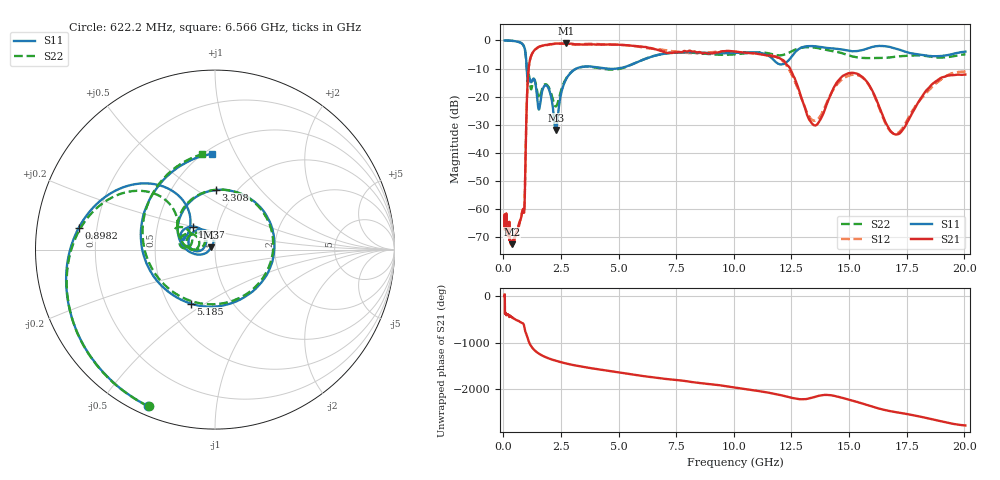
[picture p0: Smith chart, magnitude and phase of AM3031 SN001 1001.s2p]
# Hz S DB R 50
!freq MagS11 AngS11 MagS21 AngS21 MagS12 AngS12 MagS22 AngS22
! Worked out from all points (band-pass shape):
!   1601 points, 50 MHz to 20.05 GHz, reference 50 ohm
!   highest |S21| = -1.05 dB at 2.702 GHz (marker M1); lowest = -72.5 dB at 372.4 MHz (marker M2)
!   |S21| within 3 dB of the highest: 1.292 GHz to 6.925 GHz (5.633 GHz wide, 137 % of centre); 9.395 GHz to 10.15 GHz (758.8 MHz wide, 7.76 % of centre)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
!   lowest |S11| = -31.9 dB at 2.274 GHz (marker M3), VSWR 1.05, Z = 47.9 + j1.31 ohm
!   |S11| at or under -10 dB: 1.01 GHz to 3.165 GHz (2.155 GHz wide, 103 % of centre); 4.463 GHz to 4.928 GHz (464.8 MHz wide, 9.9 % of centre)
!   |S22| runs from -23.5 to 0.0 dB; largest |S21 - S12| = 0.067
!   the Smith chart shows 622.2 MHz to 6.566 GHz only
!   S11 on the Smith chart (normalised r, x): 622.2 MHz: 0.04, -0.66; 898.2 MHz: 0.13, +0.08; 1.377 GHz: 0.75, +0.20; 3.308 GHz: 0.81, +0.60; 5.185 GHz: 0.65, -0.44; 6.566 GHz: 0.54, +0.81
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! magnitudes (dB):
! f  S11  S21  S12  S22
! 50 MHz  0.0  -62.2  -67.1  0.0
! 135.9 MHz  0.0  -66.7  -66.3  0.0
! 369.6 MHz  -0.1  -72.3  -72.9  -0.1
! 372.4 MHz  -0.1  -72.5  -72.9  -0.2
! 622.2 MHz  -0.5  -67.5  -67.0  -0.5
! 898.2 MHz  -2.3  -61.1  -60.9  -2.3
! 1.005 GHz  -9.2  -24.6  -24.5  -9.7
! 1.108 GHz  -13.7  -8.9  -9.0  -12.4
! 1.377 GHz  -14.9  -3.2  -3.3  -14.6
! 1.943 GHz  -16.9  -1.5  -1.6  -16.4
! 2.274 GHz  -31.9  -1.1  -1.2  -23.5
! 2.702 GHz  -14.0  -1.1  -1.3  -13.8
! 2.722 GHz  -13.7  -1.1  -1.3  -13.5
! 3.308 GHz  -9.6  -1.4  -1.4  -9.6
! 5.185 GHz  -9.6  -1.6  -1.6  -9.8
! 6.566 GHz  -5.4  -3.1  -3.1  -5.4
! 7.402 GHz  -4.3  -4.3  -3.9  -4.3
! 11.87 GHz  -8.0  -6.0  -5.9  -5.3
! 13.53 GHz  -2.1  -30.3  -28.6  -2.6
! 15.25 GHz  -3.9  -11.7  -12.2  -5.9
! 17 GHz  -2.8  -33.4  -33.2  -5.8
! 20.05 GHz  -4.0  -12.1  -11.1  -4.9
